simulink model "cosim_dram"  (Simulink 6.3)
settings: Solver=ode45  StartTime=0.0  StopTime=1000.0  RelTol=1e-3
undefined symbols (not defined in the file or in its folder): netlist, test_dram_top
libraries: simulink x5, dram_cosim_lib x1

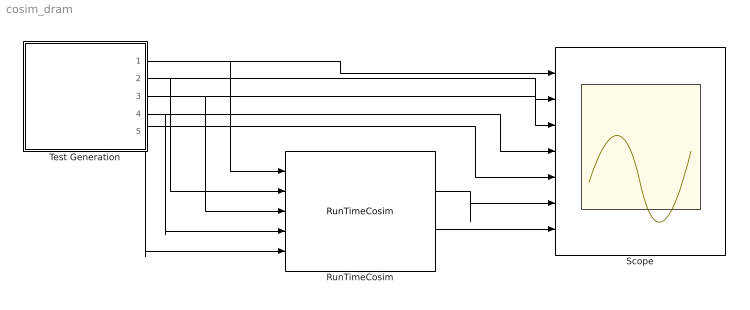
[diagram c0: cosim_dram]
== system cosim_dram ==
  RunTimeCosim : dram_cosim_lib/RunTimeCosim  index=0  bitstream=netlist/test_dram_top.bit  freq=100  single_step=on  shared=None
  Scope : Scope  NumInputPorts=7
  Test Generation : Subsystem
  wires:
  RunTimeCosim/2 -> Scope/7
  RunTimeCosim/1 -> Scope/6
  Test Generation/5(dr) -> RunTimeCosim/5, Scope/5
  Test Generation/4(dw) -> RunTimeCosim/4, Scope/4
  Test Generation/3(w) -> Scope/3, RunTimeCosim/3
  Test Generation/2(a) -> Scope/2, RunTimeCosim/2
  Test Generation/1(d) -> Scope/1, RunTimeCosim/1

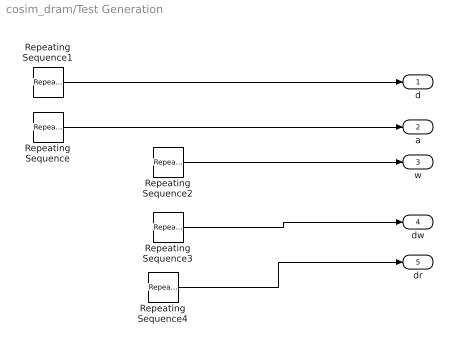
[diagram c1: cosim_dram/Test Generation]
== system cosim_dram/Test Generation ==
  Repeating Sequence : simulink/Sources/Repeating Sequence  rep_seq_t=[1:64]  rep_seq_y=[0:63]
  Repeating Sequence1 : simulink/Sources/Repeating Sequence  rep_seq_t=[1:1024]  rep_seq_y=[0:1023]
  Repeating Sequence2 : simulink/Sources/Repeating Sequence  rep_seq_t=[1:256]  rep_seq_y=[ones(1,64) zeros(1,3*64)]
  Repeating Sequence3 : simulink/Sources/Repeating Sequence  rep_seq_t=[1:1024]  rep_seq_y=[zeros(1,64) 1 zeros(1,15*64-1)]
  Repeating Sequence4 : simulink/Sources/Repeating Sequence  rep_seq_t=[1:1024]  rep_seq_y=[zeros(1,64*10) 1 zeros(1,6*64-1)]
  d : Outport
  a : Outport  Port=2
  w : Outport  Port=3
  dw : Outport  Port=4
  dr : Outport  Port=5
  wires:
  Repeating Sequence4/1 -> dr/1
  Repeating Sequence3/1 -> dw/1
  Repeating Sequence1/1 -> d/1
  Repeating Sequence2/1 -> w/1
  Repeating Sequence/1 -> a/1
